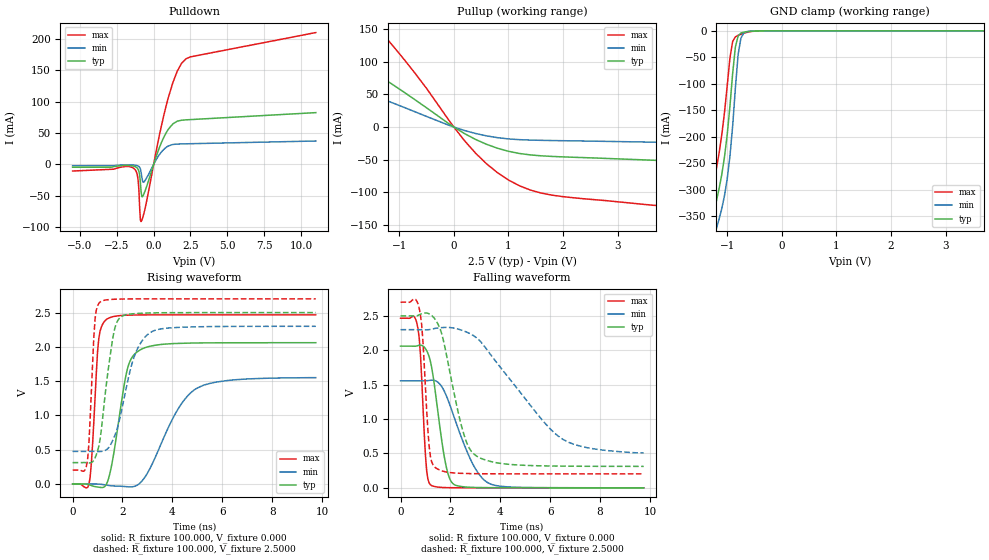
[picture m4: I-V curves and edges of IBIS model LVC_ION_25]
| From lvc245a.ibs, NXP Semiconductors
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|   Model LVC_ION_25
[Model]   LVC_ION_25
Model_type   I/O
Polarity   Non-Inverting
Enable   Active-Low
Vinl  =  0.7000V
Vinh  =  1.7000V
Vmeas =  1.25000V
Cref  = 50.0000pF
Rref  =  0.5000k
Vref  =  0.000V
C_comp   3.67pF   3.24pF   4.23pF
[Model Spec]
| Note: The input and output voltage ratings may be exceeded if the input and
|   output current ratings are observed (please refer to the data sheet)
|   Subparameter   typ   min   max
| Overshoot
S_overshoot_high   6.5   6.5   6.5   | Static overshoot
S_overshoot_low   -0.5   -0.5   -0.5
D_overshoot_high   7.2   7.2   7.2   | Dynamic overshoot
D_overshoot_low   -0.95   -0.9   -1.0
D_overshoot_time   3n   3n   3n
| Timing Thresholds
Vmeas   1.25   1.15   1.5
|Ambient temperature:   25.0000   85.0000   -40.0000
[Temperature Range]   35.0000   95.0000   -30.0000
[Voltage Range]   2.5000V   2.3000V   2.7000V
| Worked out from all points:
|   slope of the pulldown table from 0 to 0.375 V, typ, clamps not added: 14.5 ohm
|   slope of the pullup table from 0 to 0.375 V, typ, clamps not added: 20.9 ohm
|   GND clamp passes 1 mA (typ) near -0.58 V on its own axis
|   rising waveform, R_fixture 100.000, V_fixture 0.000: 20-80 % time 545ps typ, 1.29ns min, 226ps max; typ from 0 V to 2.06 V
|   rising waveform, R_fixture 100.000, V_fixture 2.5000: 20-80 % time 446ps typ, 741ps min, 193ps max; typ from 0.312 V to 2.5 V
|   falling waveform, R_fixture 100.000, V_fixture 0.000: 20-80 % time 480ps typ, 1.01ns min, 204ps max; typ from 2.06 V to 0 V
|   falling waveform, R_fixture 100.000, V_fixture 2.5000: 20-80 % time 797ps typ, 2.37ns min, 243ps max; typ from 2.5 V to 0.312 V
|Process Range   nominal   slow   fast
[Pulldown]
| voltage   I(typ)   I(min)   I(max)
-5.5V     -4.61mA    -2.142mA   -10.67mA
-1.35V    -2.944mA   -1.155mA   -6.414mA
-1.05V    -8.191mA   -2.697mA   -25.91mA
-900mV    -29.25mA   -7.337mA   -88.93mA
-850mV    -44.66mA   -12.7mA    -91.32mA
-650mV    -46.54mA   -27.94mA   -77.25mA
300mV     21.1mA     12.41mA    36.29mA
900mV     52.38mA    27.95mA    98.2mA
1.3V      64.49mA    31.72mA    130.2mA
1.9V      70.44mA    32.61mA    161.5mA
2.5V      71.41mA    32.93mA    171.6mA
11V       82.54mA    37.26mA    210.3mA
[Pullup]
| voltage   I(typ)   I(min)   I(max)
-8.7V     182.7mA    80.27mA    555.2mA
-2.9V     153.2mA    80.27mA    293.7mA
-2.3V     126.7mA    71.11mA    239.9mA
-1.5V     85.64mA    49.05mA    161.6mA
-1.3V     74.96mA    42.81mA    142.4mA
-1.1V     64.03mA    36.38mA    122.9mA
400mV     -19.05mA   -9.895mA   -40.21mA
800mV     -32.49mA   -16.27mA   -70.04mA
1.4V      -42.71mA   -19.95mA   -96.54mA
2.2V      -46.34mA   -21.15mA   -108.5mA
7.6V      -63.68mA   -28.65mA   -152.4mA
8.2V      -65.63mA   -29.49mA   -157.3mA
[GND_clamp]
| voltage   I(typ)   I(min)   I(max)
-5.5V     -4.538A    -4.57A     -4.506A
-1.35V    -431mA     -477.3mA   -376.9mA
-1.3V     -386.8mA   -433.7mA   -332mA
-1.2V     -322.6mA   -374.6mA   -261.8mA
-1.05V    -238.7mA   -311.7mA   -154.9mA
-950mV    -142.7mA   -237.3mA   -51.59mA
-900mV    -80.46mA   -179.9mA   -19.99mA
-850mV    -30.44mA   -108.2mA   -11.38mA
-800mV    -9.76mA    -44.83mA   -8.484mA
-750mV    -4.198mA   -14.39mA   -6.448mA
-700mV    -2.54mA    -4.591mA   -4.706mA
5.5V      588.5pA    6.601nA    16.7pA
[Ramp]
| variable   typ   min   max
dV/dt_r   1.236V/544.845ps   930.968mV/1.295ns   1.480V/226.521ps
dV/dt_f   1.313V/796.419ps   1.077V/2.382ns   1.498V/243.031ps
R_load = 100.000
[Rising Waveform]
R_fixture   = 100.000
V_fixture   = 0.000
V_fixture_min = 0.000
V_fixture_max = 0.000
| time   V(typ)   V(min)   V(max)
0s        31.01pV    1.698nV    3.969pV
650ps     -8.87mV    286uV      -13.24mV
750ps     -21.07mV   665.4uV    293.1mV
1.05ns    -46.06mV   -1.182mV   2.121V
1.35ns    -7.373mV   -14.87mV   2.399V
2.2ns     1.682V     -39.59mV   2.462V
2.65ns    1.942V     -1.857mV   2.466V
4.2ns     2.05V      1.076V     2.467V
5ns       2.057V     1.4V       2.467V
9.75ns    2.061V     1.551V     2.467V
[Rising Waveform]
R_fixture   = 100.000
V_fixture   = 2.5000
V_fixture_min = 2.3000
V_fixture_max = 2.7000
| time   V(typ)   V(min)   V(max)
0s        312.1mV    475.7mV    203.5mV
450ps     313.1mV    475.8mV    186.9mV
600ps     308.9mV    476mV      353.1mV
900ps     380.3mV    475.7mV    2.405V
1.1ns     647.6mV    474.2mV    2.653V
1.6ns     2.103V     630mV      2.693V
1.95ns    2.441V     1.05V      2.698V
2.5ns     2.485V     1.887V     2.7V
3.2ns     2.495V     2.226V     2.7V
9.75ns    2.5V       2.3V       2.7V
[Falling Waveform]
R_fixture   = 100.000
V_fixture   = 0.000
V_fixture_min = 0.000
V_fixture_max = 0.000
| time   V(typ)   V(min)   V(max)
0s        2.061V     1.557V     2.467V
700ps     2.068V     1.557V     2.317V
800ps     2.076V     1.556V     1.935V
1ns       2.024V     1.557V     470mV
1.2ns     1.837V     1.564V     43.64mV
1.8ns     365mV      1.37V      3.805mV
2.15ns    47.97mV    1.028V     1.727mV
2.95ns    6.077mV    311.1mV    352.7uV
3.6ns     2.748mV    56.88mV    94.24uV
9.75ns    1.768uV    445.5uV    -452.7pV
[Falling Waveform]
R_fixture   = 100.000
V_fixture   = 2.5000
V_fixture_min = 2.3000
V_fixture_max = 2.7000
| time   V(typ)   V(min)   V(max)
0s        2.5V       2.3V       2.7V
750ps     2.516V     2.3V       2.61V
900ps     2.538V     2.299V     2.125V
1.15ns    2.53V      2.301V     598.4mV
1.4ns     2.445V     2.319V     293.2mV
1.7ns     2.174V     2.331V     242.1mV
2.5ns     828mV      2.286V     209.9mV
3ns       475mV      2.195V     205.9mV
6.5ns     315.6mV    707.3mV    203.6mV
9.75ns    312.3mV    508.6mV    203.5mV
